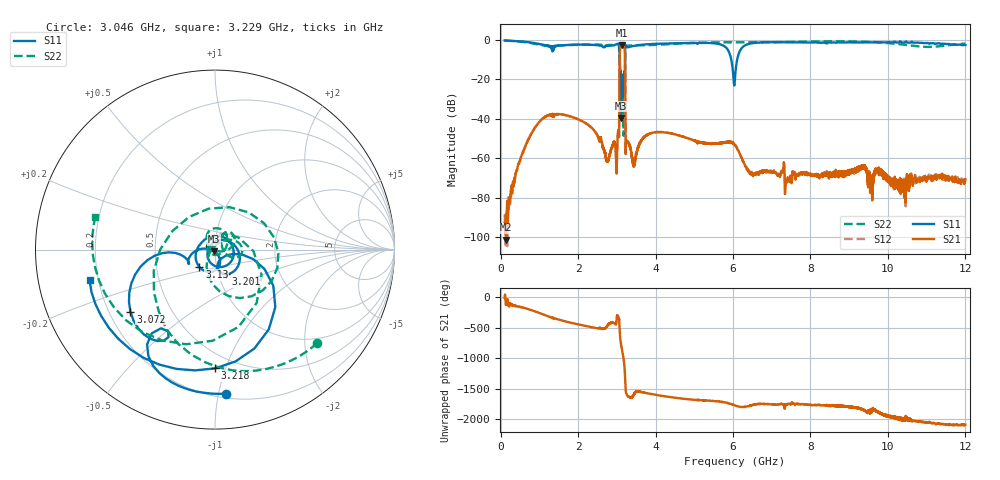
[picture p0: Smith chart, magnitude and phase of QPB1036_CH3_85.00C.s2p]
! TDS: K:\Engsetup\Winsaw\QPB1036_ALL
! Channel 1
! Ports=1 2
! seg 1=100.000000 1100.000000 101
! seg 2=1101.000000 1501.000000 401
! seg 3=1502.000000 2502.000000 101
! seg 4=2503.000000 3803.000000 1301
! seg 5=3804.000000 5004.000000 121
! seg 6=5005.000000 6005.000000 1001
! seg 7=6006.000000 8406.000000 241
! seg 8=8407.000000 10607.000000 2201
! seg 9=10608.000000 12008.000000 141
! Points=5609
! FailCode=0
! Topology=ALL_SE(12)
!VNA Cal loaded =QPB1036_ALL_85C
!PS1(V)= 5.000
!PS(mA)= 0.500
!PS2(V)= 0.630
!PS(mA)= -0.100
!PS3(V)= 1.170
!PS(mA)= 0.100
!PS4(V)= 1.170
!PS(mA)= -0.100
!Temp (C)= 85.00
# MHz S DB R 50
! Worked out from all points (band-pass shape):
!   5609 points, 100 MHz to 12.01 GHz, reference 50 ohm
!   highest |S21| = -2.68 dB at 3.126 GHz (marker M1); lowest = -101.4 dB at 140 MHz (marker M2)
!   |S21| within 3 dB of the highest: 3.08 GHz to 3.209 GHz (129 MHz wide, 4.1 % of centre)
!   lowest |S11| = -39.6 dB at 3.108 GHz (marker M3), VSWR 1.02, Z = 49.4 - j0.877 ohm
!   |S11| at or under -10 dB: 3.079 GHz to 3.212 GHz (132.7 MHz wide, 4.22 % of centre); 5.958 GHz to 6.11 GHz (152.5 MHz wide, 2.53 % of centre)
!   |S22| runs from -48.6 to -0.3 dB; largest |S21 - S12| = 0.0073
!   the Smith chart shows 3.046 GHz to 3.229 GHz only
!   S11 on the Smith chart (normalised r, x): 3.046 GHz: 0.23, -1.06; 3.072 GHz: 0.29, -0.30; 3.13 GHz: 0.83, -0.16; 3.201 GHz: 1.09, -0.31; 3.218 GHz: 0.39, -0.92; 3.229 GHz: 0.17, -0.12
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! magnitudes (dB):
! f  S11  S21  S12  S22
! 100 MHz  -0.3  -92.9  -88.6  -0.3
! 140 MHz  -0.3  -101.4  -102.8  -0.4
! 1.126 GHz  -2.7  -39.3  -39.3  -2.9
! 2.092 GHz  -2.4  -41.1  -41.2  -2.5
! 2.759 GHz  -3.1  -60.7  -60.7  -2.7
! 2.991 GHz  -2.2  -65.7  -65.0  -2.2
! 3.046 GHz  -1.9  -46.2  -46.2  -2.3
! 3.072 GHz  -4.7  -11.3  -11.3  -9.5
! 3.108 GHz  -39.6  -2.9  -2.9  -19.5
! 3.126 GHz  -17.6  -2.7  -2.7  -27.0
! 3.13 GHz  -17.8  -2.7  -2.7  -25.2
! 3.201 GHz  -16.4  -4.1  -4.1  -25.3
! 3.218 GHz  -3.6  -23.7  -23.6  -4.7
! 3.229 GHz  -2.9  -57.7  -58.1  -3.2
! 3.252 GHz  -3.5  -51.0  -51.3  -3.1
! 3.436 GHz  -3.1  -64.3  -63.4  -2.8
! 4.074 GHz  -2.0  -46.8  -46.8  -2.5
! 6.056 GHz  -18.7  -53.6  -53.5  -1.2
! 6.576 GHz  -1.5  -68.6  -67.5  -1.2
! 8.046 GHz  -1.3  -69.1  -68.3  -0.8
! 10.02 GHz  -1.1  -70.1  -70.7  -1.6
! 12.01 GHz  -2.6  -70.7  -71.2  -1.9
